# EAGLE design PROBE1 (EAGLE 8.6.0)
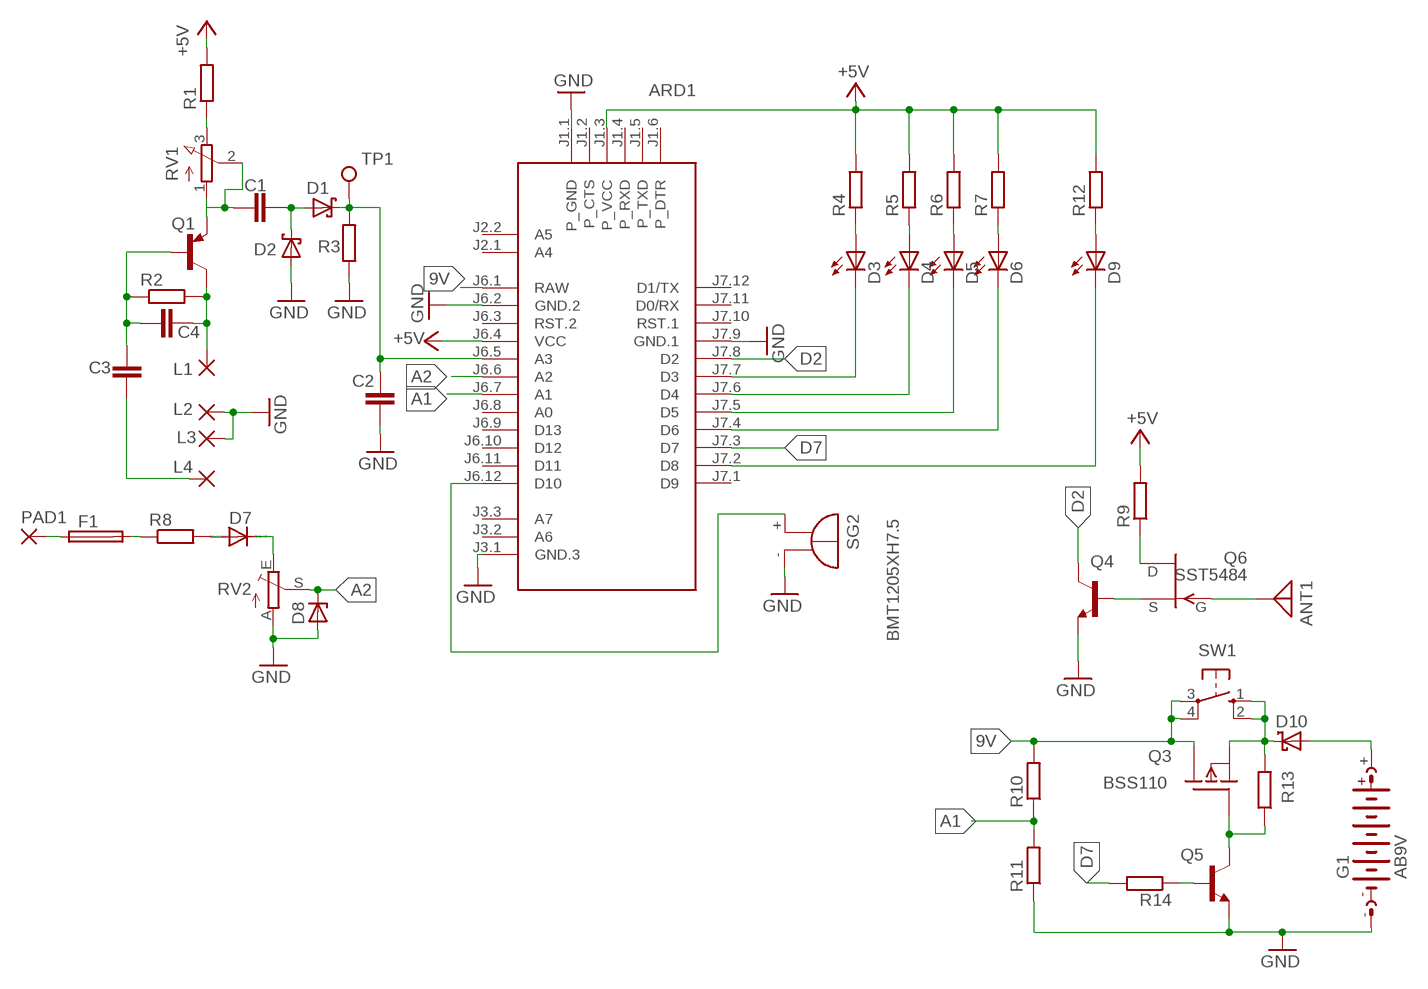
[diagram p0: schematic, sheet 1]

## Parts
ANT1  ANTENNA  [PAD-01]
ARD1  ARDUINO-PRO-MINI-3.3V  [ARDUINO-PRO-MINI]
C1  C-EUC1206  [C1206]
C2  C-EUC1206  [C1206]
C3  C-EUC1206  [C1206]
C4  C-EUC1206  [C1206]
D1  SMF5.0AT1  [SOD123FL]
D2  SMF5.0AT1  [SOD123FL]
D3  LED5MM  [LED5MM]
D4  LED5MM  [LED5MM]
D5  LED5MM  [LED5MM]
D6  LED5MM  [LED5MM]
D7  1N4004  [DO41-10]
D8  ZENER-DIODESOD80C  [SOD80C]
D9  LED5MM  [LED5MM]
D10  MBRS130LT3  [SMB]
F1  FUSESHK20Q  [SHK20Q]
G1  AB9V  [AB9V]
L1  2,15/1,0  [2,15/1,0]
L2  2,15/1,0  [2,15/1,0]
L3  2,15/1,0  [2,15/1,0]
L4  2,15/1,0  [2,15/1,0]
PAD1  3,81/1,4  [3,81/1,4]
Q1  BC327  [TO92]
Q3  BSS110  [TO92]
Q4  BC817-16LT1SMD  [SOT23-BEC]
Q5  BC337  [TO92]
Q6  SST5484  [SOT23]
R1  R-EU_R1206  [R1206]
R2  R-EU_R1206  [R1206]
R3  R-EU_R1206  [R1206]
R4  R-EU_R1206  [R1206]
R5  R-EU_R1206  [R1206]
R6  R-EU_R1206  [R1206]
R7  R-EU_R1206  [R1206]
R8  R-EU_0411/12  [0411/12]
R9  R-EU_R1206  [R1206]
R10  R-EU_R1206  [R1206]
R11  R-EU_R1206  [R1206]
R12  R-EU_R1206  [R1206]
R13  R-EU_R1206  [R1206]
R14  R-EU_R1206  [R1206]
RV1  PV09A  [PTV09]
RV2  TRIM_EU-CA6V  [CA6V]
SG2  BMT1205XH7.5  [BMT1205XH7.5]
SW1  40-XX  [B3F-40XX]
TP1  TPPAD1-13  [P1-13]

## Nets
9V: ARD1.J6.1(RAW) Q3.3(D) R10.2 SW1.3(P) SW1.4(P1)
+5V: ARD1.J1.3(P_VCC) ARD1.J6.4(VCC) R1.2 R4.2 R5.2 R6.2 R7.2 R9.2 R12.2
A1: ARD1.J6.7(A1) R10.1 R11.2
A2: ARD1.J6.6(A2) D8.C RV2.S
D2: ARD1.J7.8(D2) Q4.C
D7: ARD1.J7.3(D7) R14.2
GND: ARD1.J1.1(P_GND) ARD1.J3.1(GND.3) ARD1.J6.2(GND.2) ARD1.J7.9(GND.1) C2.2 D2.A D8.A G1.- L2.1(P) L3.1(P) Q4.E Q5.1(E) R3.1 R11.1 RV2.A SG2.-
N$1: ARD1.J7.7(D3) D3.K(C)
N$2: R1.1 RV1.3(E)
N$3: ARD1.J7.6(D4) D4.K(C)
N$4: ARD1.J7.5(D5) D5.K(C)
N$5: ARD1.J7.4(D6) D6.K(C)
N$6: ARD1.J7.2(D8) D9.K(C)
N$7: Q4.B Q6.3(S)
N$8: D3.A R4.1
N$9: D4.A R5.1
N$10: D5.A R6.1
N$11: D6.A R7.1
N$12: D9.A R12.1
N$13: ANT1.1 Q6.1(G)
N$14: Q6.2(D) R9.1
N$15: D10.A G1.+
N$16: Q3.2(G) Q5.3(C) R13.1
N$17: D10.C Q3.1(S) R13.2 SW1.1(S) SW1.2(S1)
N$18: Q5.2(B) R14.1
N$19: C1.2 Q1.1(E) RV1.1(A) RV1.2(S)
N$20: C4.1 L1.1(P) Q1.3(C) R2.2
N$21: C3.2 C4.2 Q1.2(B) R2.1
N$22: C1.1 D1.A D2.C
N$23: ARD1.J6.5(A3) C2.1 D1.C R3.2 TP1.TP
N$24: C3.1 L4.1(P)
N$25: F1.1A PAD1.1(P)
N$26: F1.2A R8.1
N$27: D7.A R8.2
N$28: D7.C RV2.E
N$29: ARD1.J6.12(D10) SG2.+
Unconnected: ARD1.J1.2(P_CTS) ARD1.J1.4(P_RXD) ARD1.J1.5(P_TXD) ARD1.J1.6(P_DTR) ARD1.J2.1(A4) ARD1.J2.2(A5) ARD1.J3.2(A6) ARD1.J3.3(A7) ARD1.J6.3(RST.2) ARD1.J6.8(A0) ARD1.J6.9(D13) ARD1.J6.10(D12) ARD1.J6.11(D11) ARD1.J7.1(D9) ARD1.J7.10(RST.1) ARD1.J7.11(D0/RX) ARD1.J7.12(D1/TX)

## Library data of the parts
ANT1 = discrete:ANTENNA: Antenna
ARD1 = diy-modules:ARDUINO-PRO-MINI-*: Arduino Pro Mini and compatible devices More details available here: https://www.arduino.cc/en/Main/ArduinoBoardProMini Click here to find device on ebay.com
C1-C4 = rcl:C-EU: CAPACITOR, European symbol
D1 D2 = diode:SMF5.0AT1: 200 W Transient Voltage Suppressor
D3-D6 D9 = led:LED: LED
D7 = diode:1N4004: DIODE
D8 = diode:ZENER-DIODE: Z-Diode
D10 = diode:MBRS130LT3: Schottky Power Rectifier
F1 = fuse:FUSE: Fuse; OC_FARNELL: unknown; OC_NEWARK: unknown
G1 = battery:AB9V: 9-V BATTERY CLIP
L1-L4 = wirepad:2,15/1,0: THROUGH-HOLE PAD
PAD1 = wirepad:3,81/1,4: THROUGH-HOLE PAD
Q1 = transistor-pnp:BC327: PNP Transistor
Q3 = transistor-fet:BSS110: P-Channel Enhancement MOSFET -50V; -0,17A; 6Ohm
Q4 = transistor-npn:BC817*: NPN Transistor
Q5 = transistor:BC337: NPN TRANSISTOR
Q6 = transistor-fet:?548*: N-Channel JFETs Source: VISHAY 2N5484.pdf Compatible: TO92 2N5245 J304 J305 U310 J308 J309 J310 TO72 2N4416 2N4416A 2N3823 2N4351 3N169 3N170 3N171 MFE3002 TO18 2N3796 2N3797 MFE825 Source: Motorola European Master Guide Pacge 3-59
R1-R14 = rcl:R-EU_: RESISTOR, European symbol
RV1 = pot:PV09A
RV2 = pot:TRIM_EU-: POTENTIOMETER
SG2 = buzzer:BMT1205XH7.5: MAGNETIC TRANSDUCER; OC_FARNELL: unknown; OC_NEWARK: unknown
SW1 = switch-omron:40-XX: OMRON SWITCH; MF: OMRON COMPONENTS USA; MPN: B3F-4000; OC_FARNELL: 176434; OC_NEWARK: 36K3105
TP1 = testpad:TP: Test pad

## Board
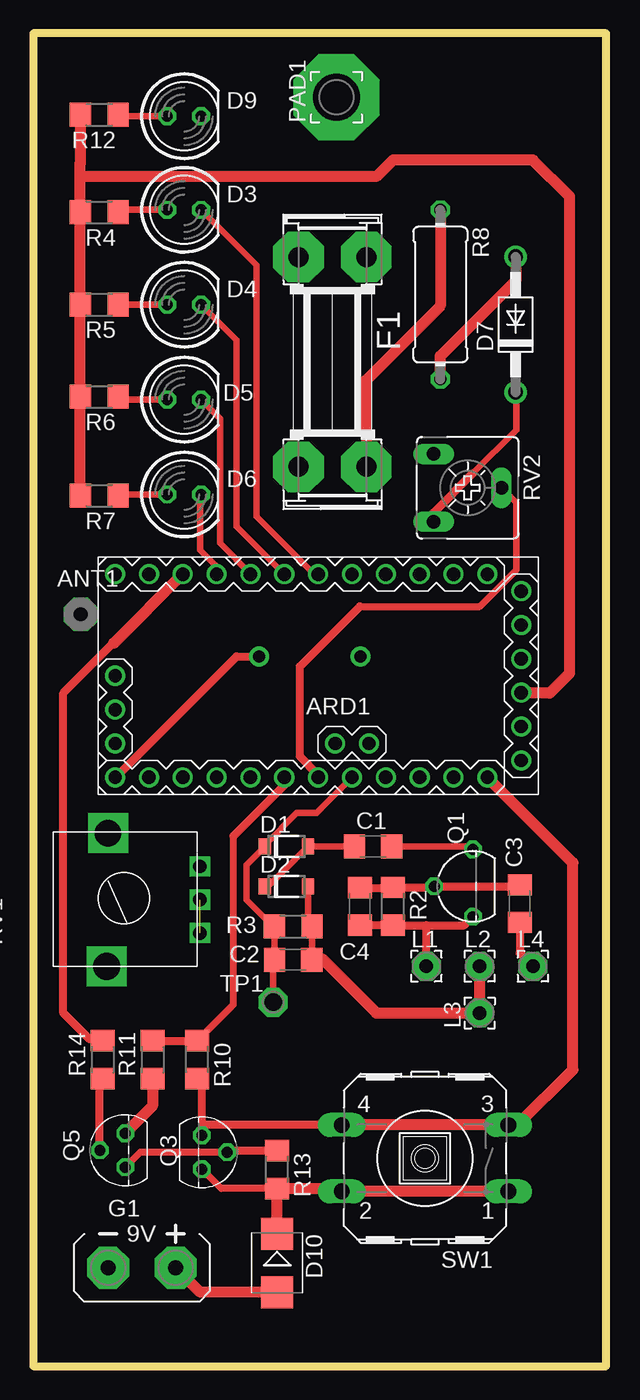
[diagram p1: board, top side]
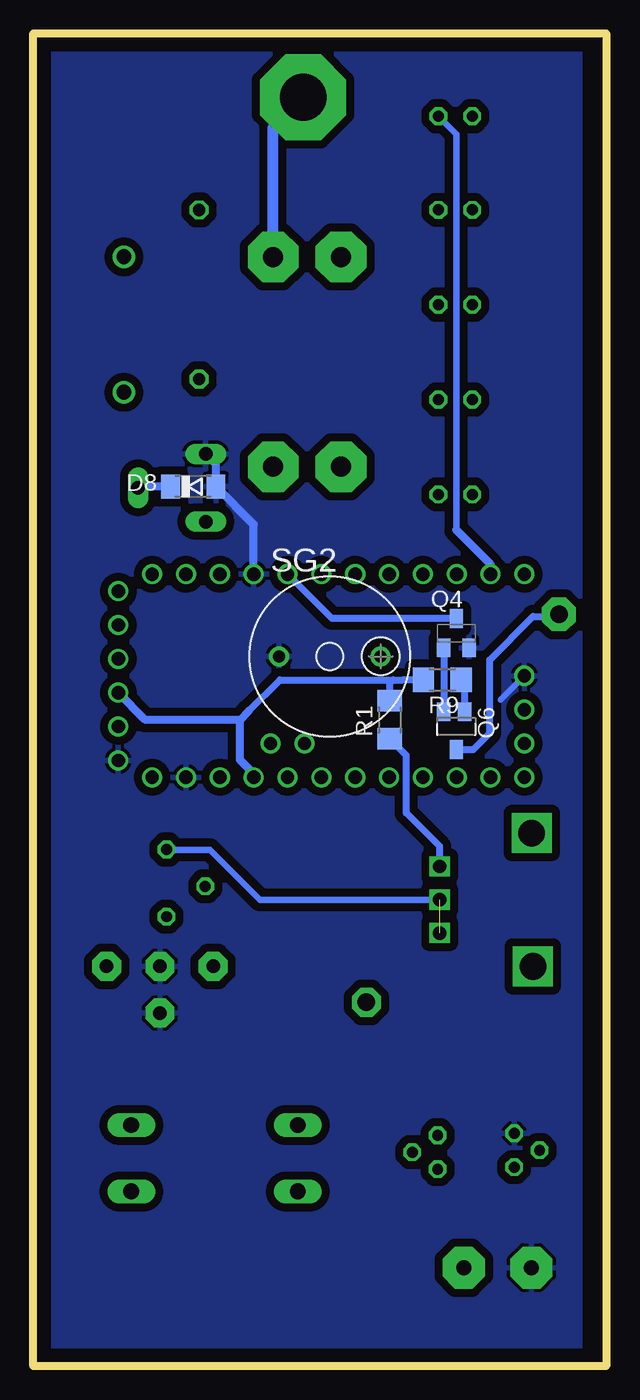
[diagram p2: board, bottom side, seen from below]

Size 43 x 100 mm. Coordinates in mm from the lower left corner, seen from the top.
Outline: 0,0 43,0 43,100 0,100 0,0
Copper layers (1*16): Top 0.035mm / dielectric 1.5mm / Bottom 0.035mm
Design rules "default": minimum track width 10mil, minimum drill 24mil, track to track 8mil, track to pad 8mil, pad to pad 8mil, via to via 8mil, smd to smd 8mil, copper to edge 40mil, drill to drill 8mil, minimum pad ring 10mil, minimum via ring 8mil, stop-mask expansion 4mil, vias tented up to drill 0mil, thermal gap 10mil

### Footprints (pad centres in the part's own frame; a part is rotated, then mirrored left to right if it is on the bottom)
PAD-01 = drill 1.321 pad 2.54 octagon: 1 0,0
ARDUINO-PRO-MINI = drill 1: J1.1 -15.24,6.35; J1.2 -15.24,3.81; J1.3 -15.24,1.27; J1.4 -15.24,-1.27; J1.5 -15.24,-3.81; J1.6 -15.24,-6.35; J2.1 -1.27,5.08; J2.2 -3.81,5.08; J3.1 15.24,0; J3.2 15.24,2.54; J3.3 15.24,5.08; J6.1 -12.7,7.62; J6.2 -10.16,7.62; J6.3 -7.62,7.62; J6.4 -5.08,7.62; J6.5 -2.54,7.62; J6.6 0,7.62; J6.7 2.54,7.62; J6.8 5.08,7.62; J6.9 7.62,7.62; J6.10 10.16,7.62; J6.11 12.7,7.62; J6.12 15.24,7.62; J7.1 15.24,-7.62; J7.2 12.7,-7.62; J7.3 10.16,-7.62; J7.4 7.62,-7.62; J7.5 5.08,-7.62; J7.6 2.54,-7.62; J7.7 0,-7.62; J7.8 -2.54,-7.62; J7.9 -5.08,-7.62; J7.10 -7.62,-7.62; J7.11 -10.16,-7.62; J7.12 -12.7,-7.62
C1206 = smd 1.6 x 1.8: 1 -1.4,0; 2 1.4,0
SOD123FL = smd 0.91 x 1.22: A 1.625,0; C -1.625,0
LED5MM = drill 0.813 octagon: A -1.27,0; K 1.27,0
DO41-10 = drill 1.118: A 5.08,0; C -5.08,0
SOD80C = smd 1.4 x 1.8: A 1.7,0; C -1.7,0
SMB = smd 2.4 x 2.4: A 2.2,0; C -2.2,0
SHK20Q = drill 1.5 pad 3.81 octagon: 1A -7.874,2.54; 1B -7.874,-2.54; 2A 7.874,2.54; 2B 7.874,-2.54
AB9V = drill 1.118 pad 3.15 octagon: + 0,2.54; - 0,-2.54
2,15/1,0 = drill 1.016 pad 2.159 octagon: 1 0,0
3,81/1,4 = drill 3.5 pad 6.452 octagon: 1 0,0
TO92 = drill 0.813 octagon: 1 2.77,0; 2 0,2.905; 3 -2.27,0
TO92' = drill 0.813 octagon: 1 1.27,0; 2 0,1.905; 3 -1.27,0
SOT23-BEC = smd 1 x 1.4: B -0.95,-1.1; C 0,1.1; E 0.95,-1.1
SOT23 = smd 1 x 1.4: 1 0,1.735; 2 -0.632,-1.1; 3 0.95,-1.1
R1206 = smd 1.6 x 1.803: 1 -1.422,0; 2 1.422,0
0411/12 = drill 0.914 octagon: 1 -6.35,0; 2 6.35,0
PTV09 = drill 1 square: 1 -2.5,0; 2 0,0; 3 2.5,0 | drill 2 square: P$4 -5,7; P$5 5,6.9
CA6V = drill 1.016 long: A -2.54,-2.54; E 2.54,-2.54; S 0,2.54
BMT1205XH7.5 = drill 0.9 pad 1.5: + 3.8,0; - -3.8,0
B3F-40XX = drill 1.194 long: 1 -6.248,2.489; 2 6.248,2.489; 3 -6.248,-2.489; 4 6.248,-2.489
P1-13 = drill 1.321 pad 2.159 octagon: TP 0,0

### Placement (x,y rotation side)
ANT1  3.55,56.41 0 top
ARD1  21.38,51.8 180 top
C1  25.5,39 0 top
C2  19.5,30.5 0 top
C3  36.5,34.7 90 top
C4  24.5,34.5 90 top
D1  19,39 0 top
D2  19,36 0 top
D3  11.32,86.76 0 top
D4  11.32,79.64 0 top
D5  11.32,72.52 0 top
D6  11.32,65.4 0 top
D7  36.2,78.15 90 top
D8  31,66 0 bottom
D9  11.32,93.78 0 top
D10  18.3,7.75 270 top
F1  22.45,75.35 270 top
G1  8.15,7.39 270 top
L1  29.5,30 0 top
L2  33.5,30 0 top
L3  33.5,26.5 90 top
L4  37.5,30 0 top
PAD1  22.75,95.2 90 top
Q1  33,36 90 top
Q3  BSS110  [TO92']  12.65,16.05 270 top
Q4  11.25,55 0 bottom
Q5  BC337  [TO92']  6.9,16.2 90 top
Q6  11.25,48 180 bottom
R1  16.25,48.5 90 bottom
R2  27,34.5 270 top
R3  19.5,33 180 top
R4  4.95,86.57 180 top
R5  4.95,79.65 180 top
R6  4.95,72.73 180 top
R7  4.95,65.31 180 top
R8  30.55,80.4 270 top
R9  12.3,51.5 180 bottom
R10  12.3,23 270 top
R11  8.95,23 90 top
R12  4.95,93.89 180 top
R13  18.3,14.75 270 top
R14  5.2,23 90 top
RV1  12.5,35 90 top
RV2  32.6,65.9 270 top
SG2  20.75,53.25 0 bottom
SW1  29.4,15.6 180 top
TP1  18,27.3 0 top

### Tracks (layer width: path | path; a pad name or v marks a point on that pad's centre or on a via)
9V
  Top 0.61: Q3.3 12.65,18 | 12.65,18 12.65,21.23 R10.2 | SW1.4 12.74,18.09 12.65,18
  Top 0.813: SW1.4 SW1.3 36.34,18.09 40.5,22.25 40.5,37.76 ARD1.J6.1
+5V
  Top 0.813: R12.2 3.53,90.28 3.5,90.25 3.53,90.22 3.53,89.5 | ARD1.J1.3 36.65,50.5 38.75,50.5 40.25,52 40.25,87.75 37.5,90.5 27,90.5 25.75,89.25 3.78,89.25 3.53,89.5 | 3.53,89.5 R4.2 R5.2 R6.2 R7.2
  Bottom 0.51: 26.83,49.17 24.5,51.5 16,51.5 | 16,51.5 15.25,51.5 R9.2 | R1.2 16.25,51.25 16,51.5
  Bottom 0.61: 27.5,48.5 34.59,48.5 ARD1.J1.3 | ARD1.J6.4 26.46,44.46 27.5,45.5 27.5,48.5 | 26.83,49.17 27.5,48.5
A1
  Top 0.51: 15,39.75 15,27.12 R10.1
  Top 0.61: R11.2 R10.1 | ARD1.J6.7 18.84,43.59 15,39.75
A2
  Top 0.5: 36.25,59.75 36.25,64.79 RV2.S
  Top 0.51: 24.5,57 33.5,57 36.25,59.75
  Top 0.61: ARD1.J6.6 21.38,44.37 20,45.75 20,52.5 24.5,57
  Bottom 0.61: D8.C 35.04,66 RV2.S
D2
  Bottom 0.51: Q4.C 20.6,56.1 ARD1.J7.8
D7
  Top 0.61: 5.2,24.55 4.2,24.55 2.25,26.5 2.25,50.5 6,54.25
  Top 0.813: R14.2 5.2,24.55 | 6,54.25 6.05,54.25 ARD1.J7.3
GND
  Top 0.5: D2.A 20.62,33.3 R3.1 20.92,30.52 C2.2
  Top 0.813: 20.92,30.52 21.73,30.52 25.75,26.5 L3.1 L2.1 | R11.1 8.95,19.52 Q5.1
  Bottom 0.406: 7.94,50 ARD1.J3.1
  Bottom 0.61: ARD1.J7.9 26.46,63.16 D8.A 29.3,67.68 RV2.A
  pour Bottom (isolate 0.61): 2,99 42,99 42,1 2,1
N$1
  Top 0.5: ARD1.J7.7 21.08,59.42 16.75,63.75 16.75,82.6 D3.K
N$2
  Bottom 0.51: R1.1 15,45.83 15,41.5 12.5,39 RV1.3
N$3
  Top 0.5: ARD1.J7.6 15.25,63 15.25,76.98 D4.K
N$4
  Top 0.5: ARD1.J7.5 16.3,59.45 14,61.75 14,71.11 D5.K
N$5
  Top 0.5: ARD1.J7.4 13.76,59.99 12.5,61.25 12.5,65.31 D6.K
N$6
  Bottom 0.5: 11.25,62.75 11.25,92.44 D9.K
  Bottom 0.61: ARD1.J7.2 8.68,60.18 11.25,62.75
N$7
  Bottom 0.51: Q4.B Q6.3
N$8
  Top 0.5: D3.A 6.56,86.76 R4.1
N$9
  Top 0.5: D4.A 6.38,79.64 R5.1
N$10
  Top 0.5: D5.A 6.58,72.52 R6.1
N$11
  Top 0.5: D6.A 6.46,65.4 R7.1
N$12
  Top 0.5: D9.A 6.48,93.78 R12.1
N$13
  Bottom 0.51: Q6.1 11.23,46.25 10,46.25 8.75,47.5 8.75,53 5.5,56.25 3.89,56.25 ANT1.1
N$14
  Bottom 0.51: Q6.2 10.62,51.24 R9.1
N$15
  Top 0.813: D10.A 12.53,5.55 G1.+
N$16
  Top 0.51: Q3.2 8.02,16.05 Q5.3
  Top 0.61: R13.1 14.68,16.17 Q3.2
N$17
  Top 0.51: R13.2 14.1,13.33 Q3.1
  Top 0.813: SW1.1 SW1.2 22.93,13.33 R13.2 D10.C
N$18
  Top 0.61: Q5.2 5,21.37 R14.1
N$19  (1 unrouted)
  Top 0.5: C1.2 32.77,39 Q1.1
  Bottom 0.5: RV1.2 26,35 29.75,38.75 32.98,38.75 Q1.1
N$20
  Top 0.61: C4.1 24.52,33.08 R2.2 29.5,33.08 | 29.5,33.08 32.35,33.08 Q1.3 | L1.1 29.5,33.08
N$21
  Top 0.61: C3.2 36.4,36 Q1.2 30.02,35.92 R2.1 26.98,35.9 C4.2
N$22
  Top 0.5: D2.C 17.62,36 D1.A C1.1
N$23
  Top 0.5: TP1.TP 18,30.4 C2.1 18.1,32.98 R3.2 18,33 16,35 16,37.62 D1.C 17.38,39.12 19.75,41.5 21.24,41.5 ARD1.J6.5
N$24
  Top 0.61: C3.1 36.5,31 L4.1
N$25
  Bottom 0.813: F1.1A 24.99,92.96 PAD1.1
N$26
  Top 0.813: R8.1 30.55,79.55 25,74 F1.2A
N$27
  Top 0.813: R8.2 30.55,75.8 36.25,81.5 36.25,83.18 D7.A
N$28
  Top 0.5: 33,67 36.25,70.25 36.25,73.02 D7.C
  Top 0.61: RV2.E 30.06,64.06 33,67
N$29
  Top 0.61: ARD1.J6.12 6.18,44.18 15.25,53.25 SG2.+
